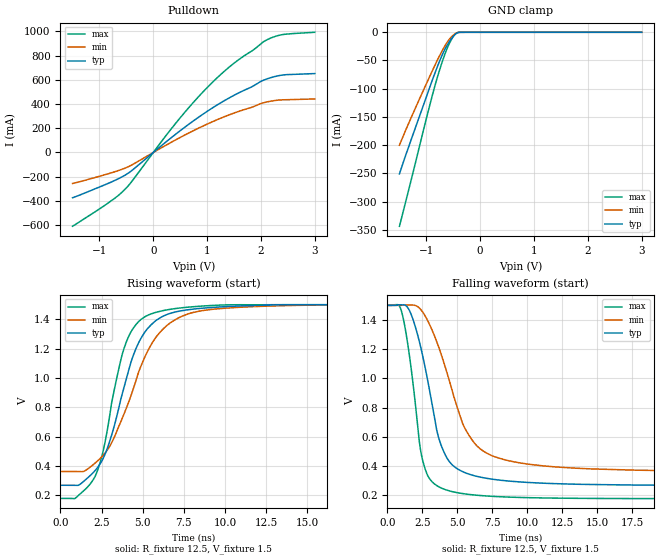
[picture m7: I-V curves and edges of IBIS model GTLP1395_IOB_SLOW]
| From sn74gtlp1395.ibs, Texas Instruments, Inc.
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[Model]   GTLP1395_IOB_SLOW
Model_type  I/O_open_drain
Vinl = 0.95
Vinh = 1.05
Enable   Active-Low
Vref =   1.5
Rref =   12.5
Cref =   30p
Vmeas =   1.0
| variable   typ   min   max
C_comp   7.53pF   6.02pF   8.49pF
| C_pulldown   9.18pF   5.44pF   15.50pF
| C_tri-state   7.53pF   6.02pF   8.49pF
[Temperature Range]   40   100   -40
| Ambient temperature   25   85   -40
[Voltage range]   1.5   1.5   1.5
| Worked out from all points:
|   slope of the pulldown table from 0 to 0.225 V, typ, clamps not added: 2.7 ohm
|   GND clamp passes 1 mA (typ) near -0.42 V on its own axis
|   rising waveform, R_fixture 12.5, V_fixture 1.5: 20-80 % time 1.98ns typ, 2.52ns min, 1.51ns max; typ from 0.267 V to 1.5 V
|   falling waveform, R_fixture 12.5, V_fixture 1.5: 20-80 % time 1.68ns typ, 2.53ns min, 1.06ns max; typ from 1.5 V to 0.268 V
[GND Clamp]
| GTLP1395_IOB_SLOW
|   Voltage   I(typ)   I(min)   I(max)
-1.5V     -251mA     -200.2mA   -343.9mA
-1.325V   -202mA     -160.6mA   -278.1mA
-980mV    -109.1mA   -87.16mA   -145.5mA
-880mV    -82.51mA   -66.47mA   -108.8mA
-800mV    -62.2mA    -50.39mA   -81.3mA
-695mV    -38.08mA   -30.87mA   -49.54mA
-610mV    -22.36mA   -17.3mA    -27.87mA
-525mV    -10.04mA   -7.253mA   -11.29mA
-450mV    -2.617mA   -1.767mA   -2.187mA
-410mV    -522.4uA   -344.4uA   -180.8uA
-355mV    -26.7uA    -53.58uA   -21.94uA
3V        1.146nA    5.211nA    8.435nA
[Pulldown]
| GTLP1395_IOB_SLOW
|   Voltage   I(typ)   I(min)   I(max)
-1.5V     -373.9mA   -256.1mA   -609.8mA
-835mV    -254.7mA   -175.4mA   -415.9mA
-530mV    -188.7mA   -129.9mA   -306.1mA
-405mV    -151.2mA   -104.3mA   -242.4mA
280mV     103.2mA    71.14mA    164.8mA
640mV     227.1mA    156.7mA    360.7mA
1.065V    358.5mA    247.4mA    565mA
1.465V    464.1mA    320.2mA    725.2mA
2.04V     595.6mA    409.6mA    912.6mA
2.205V    621.2mA    425.6mA    949.4mA
2.435V    641.6mA    435.6mA    976.1mA
3V        652.1mA    442.2mA    993.1mA
[Ramp]
| GTLP1395_IOB_SLOW
| variable   typ   min   max
dV/dt_r   0.74/2.04E-09   0.68/2.59E-09   0.79/1.53E-09
dV/dt_f   0.74/1.69E-09   0.68/2.54E-09   0.80/1.07E-09
R_load = 12.5
[Rising Waveform]
| GTLP1395_IOB_SLOW
R_fixture =   12.5
C_fixture =   0
L_fixture =   0
V_fixture =   1.5
V_fixture_min = 1.5
V_fixture_max = 1.5
|   Time   V(typ)   V(min)   V(max)
0s        267.4mV    361.4mV    177.7mV
885ps     267.2mV    361.3mV    177.8mV
2.09ns    365.9mV    417.4mV    324.4mV
2.885ns   531.2mV    514.4mV    668.3mV
3.855ns   932.5mV    751.9mV    1.198V
4.51ns    1.178V     954.4mV    1.352V
5.255ns   1.332V     1.173V     1.425V
6.67ns    1.441V     1.376V     1.468V
8.805ns   1.478V     1.462V     1.492V
25ns      1.5V       1.5V       1.5V
[Falling Waveform]
| GTLP1395_IOB_SLOW
R_fixture =   12.5
C_fixture =   0
L_fixture =   0
V_fixture =   1.5
V_fixture_min = 1.5
V_fixture_max = 1.5
|   Time   V(typ)   V(min)   V(max)
0s        1.5V       1.5V       1.5V
950ps     1.504V     1.5V       1.479V
1.725ns   1.433V     1.502V     1.054V
2.495ns   1.17V      1.459V     453.4mV
2.945ns   957.7mV    1.384V     326.2mV
3.675ns   594mV      1.215V     259.5mV
4.415ns   434.1mV    991.9mV    231.8mV
5.515ns   357.4mV    665.9mV    211.1mV
7.495ns   311.4mV    471.4mV    194mV
25ns      268.3mV    365mV      177.8mV
